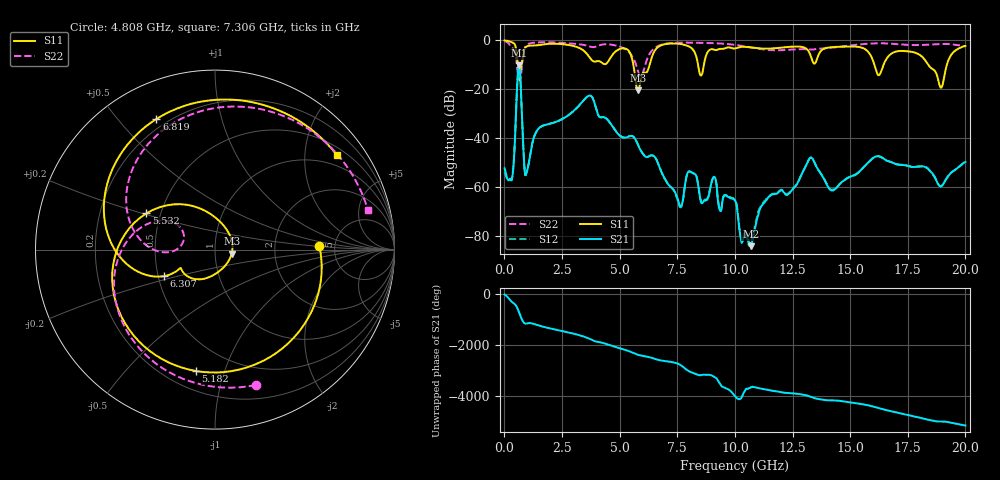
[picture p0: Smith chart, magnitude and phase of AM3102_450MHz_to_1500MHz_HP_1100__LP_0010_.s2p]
!Agilent Technologies,E8364B,MY43040894,A.07.50.67
!Agilent E8364B: A.07.50.67
!Date: Thursday, January 11, 2018 06:32:18
!Correction: S11(Full 2 Port(1,2))
!S21(Full 2 Port(1,2))
!S12(Full 2 Port(1,2))
!S22(Full 2 Port(1,2))
!S2P File: Measurements: S11, S21, S12, S22:
# Hz S  dB  R 50
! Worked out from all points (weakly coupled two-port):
!   1601 points, 10 MHz to 20 GHz, reference 50 ohm
!   highest |S21| = -10.17 dB at 634.7 MHz (marker M1); lowest = -84.1 dB at 10.69 GHz (marker M2)
!   lowest |S11| = -20.4 dB at 5.795 GHz (marker M3), VSWR 1.21, Z = 60.2 - j2.68 ohm
!   |S11| at or under -10 dB: 5.595 GHz to 6.302 GHz (707 MHz wide, 11.9 % of centre); 16.05 GHz to 16.45 GHz (400.5 MHz wide, 2.46 % of centre); 18.39 GHz to 19.2 GHz (810.3 MHz wide, 4.31 % of centre)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
!   |S22| runs from -16.3 to -0.4 dB; largest |S21 - S12| = 0.00092
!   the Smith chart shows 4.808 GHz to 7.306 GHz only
!   S11 on the Smith chart (normalised r, x): 4.808 GHz: 3.76, +0.25; 5.182 GHz: 0.32, -0.81; 5.532 GHz: 0.42, +0.21; 6.307 GHz: 0.54, -0.18; 6.819 GHz: 0.16, +0.64; 7.306 GHz: 0.69, +2.78
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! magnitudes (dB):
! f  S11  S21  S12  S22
! 10 MHz  -0.1  -52.3  -53.9  -0.4
! 334.8 MHz  -0.9  -56.4  -56.3  -3.1
! 634.7 MHz  -11.8  -10.2  -10.2  -15.9
! 959.5 MHz  -2.6  -54.2  -54.1  -2.0
! 1.472 GHz  -2.0  -36.2  -36.2  -0.9
! 3.346 GHz  -3.6  -25.5  -25.5  -1.7
! 4.808 GHz  -4.7  -36.8  -36.8  -2.1
! 5.182 GHz  -3.3  -39.8  -39.7  -3.3
! 5.532 GHz  -7.3  -39.1  -39.1  -6.4
! 5.795 GHz  -20.4  -42.7  -42.7  -12.6
! 6.307 GHz  -9.9  -47.2  -47.2  -5.5
! 6.682 GHz  -2.7  -50.7  -50.6  -2.3
! 6.819 GHz  -2.0  -54.0  -53.9  -1.8
! 7.306 GHz  -1.3  -60.8  -60.7  -1.1
! 8.531 GHz  -14.4  -66.0  -65.9  -1.0
! 10.01 GHz  -3.4  -65.5  -65.3  -1.9
! 10.69 GHz  -2.9  -84.1  -82.5  -2.9
! 13.34 GHz  -7.8  -48.1  -48.1  -3.8
! 14.22 GHz  -2.8  -61.3  -61.0  -3.0
! 16.68 GHz  -6.4  -49.4  -49.5  -1.3
! 18.94 GHz  -19.4  -59.8  -59.6  -1.5
! 20 GHz  -2.3  -49.7  -49.6  -2.4
